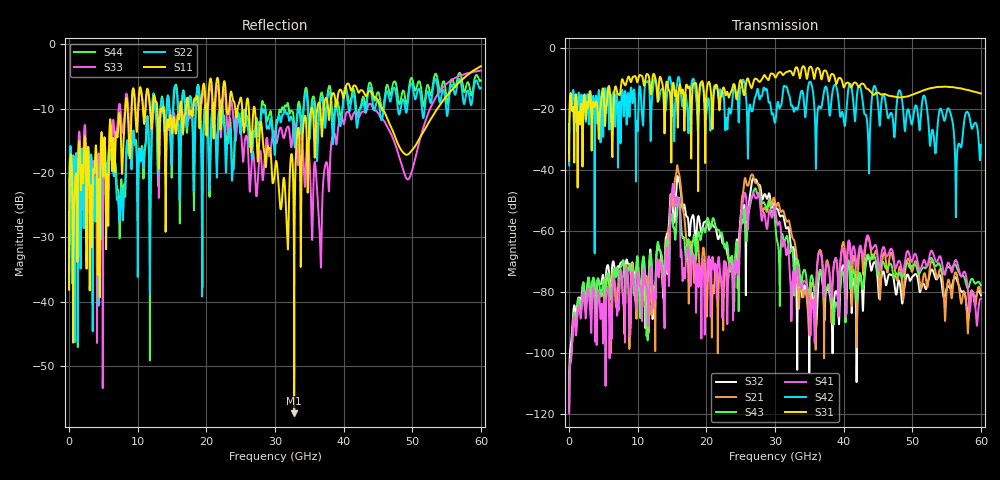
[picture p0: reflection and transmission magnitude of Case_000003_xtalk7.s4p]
! Info: Touchstone file created by circ.  Input file=CasetestDOE_NRZ_template_000003.circ
# Hz S RI R 50
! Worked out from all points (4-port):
!   6000 points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, 10 MHz to 60 GHz, reference 50 ohm
!   strongest paths, dB at 10 MHz, 15.01 GHz, 30.01 GHz, 45.01 GHz, 60 GHz:
!     S31: -36.9, -15.9, -9.7, -14.7, -15.0
!     S42: -38.6, -14.8, -24.6, -18.3, -31.8
!     S41: -119.8, -47.3, -52.6, -69.7, -82.3
!     S43: -119.2, -54.5, -57.0, -74.4, -77.9
!     S21: -119.2, -48.0, -50.6, -70.0, -80.4
!     S32: -116.8, -49.6, -51.4, -77.6, -81.2
!   lowest |S11| = -57.3 dB at 32.8 GHz (marker M1), VSWR 1.00, Z = 49.9 + j0.0677 ohm
!   |S11| at or under -10 dB: start of sweep to 8.203 GHz; 27.05 GHz to 35.32 GHz (8.271 GHz wide, 26.5 % of centre); 45.61 GHz to 53.67 GHz (8.067 GHz wide, 16.3 % of centre)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
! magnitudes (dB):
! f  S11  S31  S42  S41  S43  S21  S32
! 10 MHz  -38.1  -36.9  -38.6  -119.8  -119.2  -119.2  -116.8
! 12.32 GHz  -8.4  -8.5  -11.7  -83.0  -82.6  -78.3  -82.0
! 15.81 GHz  -11.0  -23.9  -10.6  -49.0  -52.4  -38.8  -42.1
! 20.96 GHz  -11.5  -21.7  -17.5  -69.1  -55.9  -77.9  -58.2
! 26.62 GHz  -15.3  -13.2  -20.8  -49.2  -49.4  -41.6  -44.1
! 32.8 GHz  -57.3  -8.2  -20.9  -75.5  -80.5  -63.1  -66.6
! 60 GHz  -3.4  -15.0  -31.8  -82.3  -77.9  -80.4  -81.2
